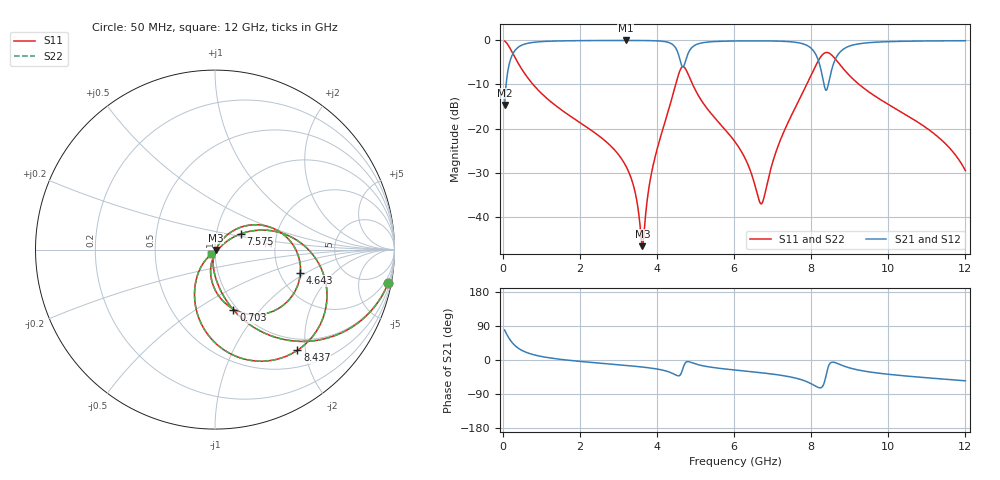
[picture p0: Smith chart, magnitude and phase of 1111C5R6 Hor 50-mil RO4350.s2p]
# GHz S MA R 50
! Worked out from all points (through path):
!   11951 points, 50 MHz to 12 GHz, reference 50 ohm
!   highest |S21| = -0.03 dB at 3.196 GHz (marker M1); lowest = -14.7 dB at 50 MHz (marker M2)
!   group delay of S21, straight-line fit = 15.6 ps
!   lowest |S11| = -46.6 dB at 3.624 GHz (marker M3), VSWR 1.01, Z = 50.4 - j0.186 ohm
!   |S11| at or under -10 dB: 788.2 MHz to 4.486 GHz (3.698 GHz wide, 140 % of centre); 4.927 GHz to 7.884 GHz (2.957 GHz wide, 46.2 % of centre); 9.244 GHz to end of sweep
!   |S22| runs from -46.6 to -0.2 dB; largest |S21 - S12| = 0
!   S11 on the Smith chart (normalised r, x): 50 MHz: 1, -10; 703 MHz: 0.96, -0.73; 4.643 GHz: 2.59, -0.89; 7.575 GHz: 1.31, +0.24; 8.437 GHz: 0.78, -1.85; 12 GHz: 0.96, -0.05
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0.05  0.9828 -10.9  0.1847 79.1  0.1847 79.1  0.9828 -10.9
0.253  0.7241 -44.9  0.6892 45.1  0.6892 45.1  0.7241 -44.9
0.703  0.3509 -73.0  0.9356 16.9  0.9356 16.9  0.3509 -73.0
2.042  0.114 -93.4  0.992 -4.0  0.992 -4.0  0.114 -93.4
3.196  0.03762 -100.5  0.9966 -14.3  0.9966 -14.3  0.03762 -100.5
3.425  0.01984 -96.8  0.9963 -16.5  0.9963 -16.5  0.01984 -96.8
3.624  0.00466 -23.3  0.9951 -18.6  0.9951 -18.6  0.00466 -23.3
3.821  0.02546 52.7  0.9923 -21.0  0.9923 -21.0  0.02546 52.7
4.034  0.06512 53.9  0.9845 -24.3  0.9845 -24.3  0.06512 53.9
4.471  0.299 26.9  0.8382 -38.7  0.8382 -38.7  0.299 26.9
4.643  0.4932 -15.3  0.517 -31.8  0.517 -31.8  0.4932 -15.3
4.78  0.4418 -54.9  0.6585 -4.5  0.6585 -4.5  0.4418 -54.9
5.025  0.2594 -85.3  0.8973 -11.1  0.8973 -11.1  0.2594 -85.3
6.025  0.0709 -104.7  0.9827 -26.5  0.9827 -26.5  0.0709 -104.7
6.713  0.0141 -31.7  0.9855 -33.7  0.9855 -33.7  0.0141 -31.7
7.575  0.1683 31.4  0.9525 -47.2  0.9525 -47.2  0.1683 31.4
8.017  0.4189 10.5  0.7993 -63.5  0.7993 -63.5  0.4189 10.5
8.264  0.664 -20.2  0.4449 -72.6  0.4449 -72.6  0.664 -20.2
8.437  0.725 -50.7  0.3056 -19.7  0.3056 -19.7  0.725 -50.7
8.883  0.4505 -97.4  0.8184 -17.3  0.8184 -17.3  0.4505 -97.4
10.009  0.1872 -123.0  0.9663 -37.8  0.9663 -37.8  0.1872 -123.0
12  0.03345 -128.5  0.9895 -54.9  0.9895 -54.9  0.03345 -128.5
